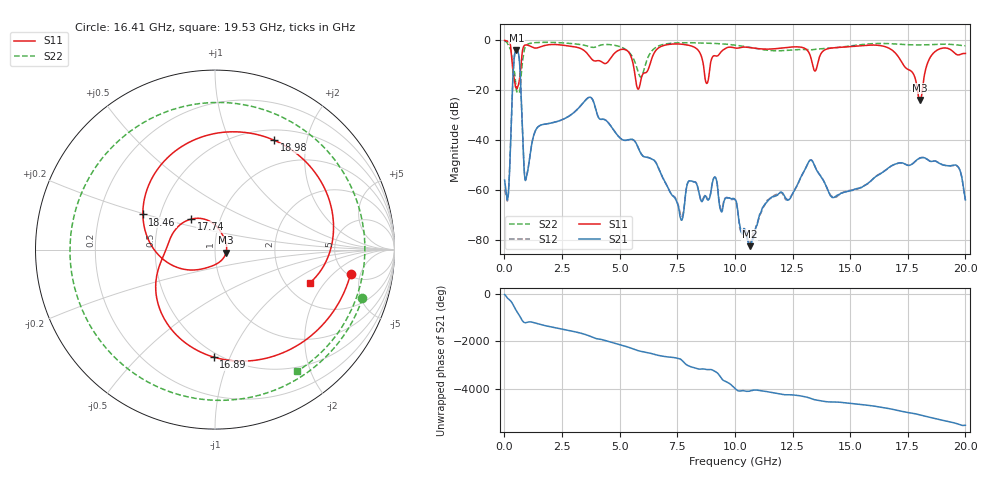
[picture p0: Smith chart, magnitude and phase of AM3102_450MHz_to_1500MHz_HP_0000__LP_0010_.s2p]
!Agilent Technologies,E8364B,MY43040894,A.07.50.67
!Agilent E8364B: A.07.50.67
!Date: Thursday, January 11, 2018 05:14:17
!Correction: S11(Full 2 Port(1,2))
!S21(Full 2 Port(1,2))
!S12(Full 2 Port(1,2))
!S22(Full 2 Port(1,2))
!S2P File: Measurements: S11, S21, S12, S22:
# Hz S  dB  R 50
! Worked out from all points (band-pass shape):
!   1601 points, 10 MHz to 20 GHz, reference 50 ohm
!   highest |S21| = -3.87 dB at 522.2 MHz (marker M1); lowest = -82.4 dB at 10.64 GHz (marker M2)
!   |S21| within 3 dB of the highest: 428.9 MHz to 638.6 MHz (209.7 MHz wide, 39.3 % of centre)
!   lowest |S11| = -23.9 dB at 18.03 GHz (marker M3), VSWR 1.14, Z = 56.6 - j1.89 ohm
!   |S11| at or under -10 dB: 347.4 MHz to 722.3 MHz (374.9 MHz wide, 70.1 % of centre); 5.597 GHz to 6.303 GHz (705.9 MHz wide, 11.9 % of centre); 17.32 GHz to 18.33 GHz (1.005 GHz wide, 5.64 % of centre)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
!   |S22| runs from -21.2 to -0.3 dB; largest |S21 - S12| = 0.0019
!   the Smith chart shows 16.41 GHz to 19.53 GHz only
!   S11 on the Smith chart (normalised r, x): 16.41 GHz: 5.29, -3.47; 16.89 GHz: 0.47, -0.87; 17.74 GHz: 0.73, +0.26; 18.46 GHz: 0.40, +0.20; 18.98 GHz: 0.63, +1.49; 19.53 GHz: 2.68, -1.44
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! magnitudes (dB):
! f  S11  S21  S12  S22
! 10 MHz  -0.1  -56.0  -59.8  -0.3
! 172.4 MHz  -0.6  -61.6  -61.5  -2.0
! 522.2 MHz  -18.9  -3.9  -3.9  -20.0
! 947 MHz  -1.9  -55.2  -55.1  -2.0
! 3.346 GHz  -3.4  -25.8  -25.8  -1.8
! 5.807 GHz  -19.6  -43.0  -43.0  -12.8
! 6.682 GHz  -3.1  -51.1  -51.1  -2.3
! 7.681 GHz  -1.6  -72.1  -70.8  -1.0
! 8.781 GHz  -17.3  -63.3  -63.0  -1.1
! 10.01 GHz  -3.1  -63.7  -63.8  -1.9
! 10.64 GHz  -2.9  -82.4  -80.8  -2.8
! 13.34 GHz  -8.6  -48.1  -48.1  -3.8
! 14.25 GHz  -3.0  -62.9  -62.8  -3.1
! 16.41 GHz  -2.3  -52.9  -52.7  -1.3
! 16.68 GHz  -3.1  -51.0  -51.0  -1.3
! 16.89 GHz  -4.4  -49.9  -49.9  -1.4
! 17.74 GHz  -13.4  -49.2  -49.2  -1.8
! 18.03 GHz  -23.9  -47.1  -47.1  -1.9
! 18.46 GHz  -7.0  -48.4  -48.3  -1.7
! 18.98 GHz  -3.2  -49.8  -49.7  -1.6
! 19.53 GHz  -5.0  -50.0  -50.1  -1.7
! 20 GHz  -5.3  -63.9  -64.0  -2.2
